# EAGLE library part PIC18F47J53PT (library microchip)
PIC18F47J53 Family High-Performance USB Microcontrollers with nanoWatt XLP Technology Source: Data sheet
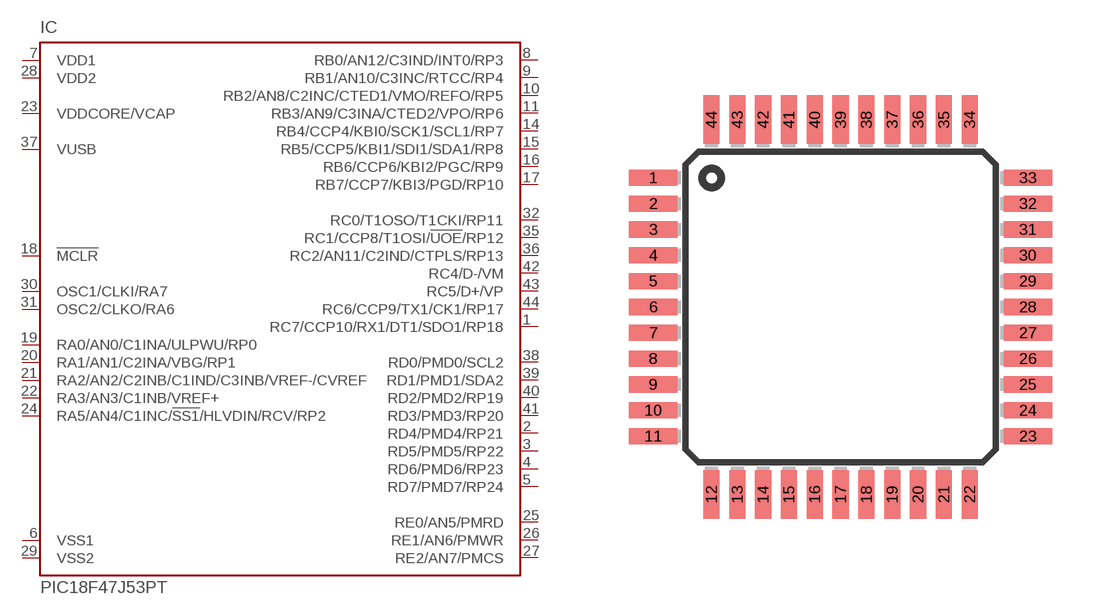
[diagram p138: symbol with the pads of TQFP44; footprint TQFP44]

Designator prefix IC

## PIC18F47J53PT (MPN: PIC18F47J53-I/PT; OC_FARNELL: 1815001; OC_NEWARK: 63R7856)  [TQFP44]
1  RC7/CCP10/RX1/DT1/SDO1/RP18
2  RD4/PMD4/RP21
3  RD5/PMD5/RP22
4  RD6/PMD6/RP23
5  RD7/PMD7/RP24
6  VSS1  in
7  VDD1  in
8  RB0/AN12/C3IND/INT0/RP3
9  RB1/AN10/C3INC/RTCC/RP4
10  RB2/AN8/C2INC/CTED1/VMO/REFO/RP5
11  RB3/AN9/C3INA/CTED2/VPO/RP6
14  RB4/CCP4/KBI0/SCK1/SCL1/RP7
15  RB5/CCP5/KBI1/SDI1/SDA1/RP8
16  RB6/CCP6/KBI2/PGC/RP9
17  RB7/CCP7/KBI3/PGD/RP10
18  !MCLR  in
19  RA0/AN0/C1INA/ULPWU/RP0
20  RA1/AN1/C2INA/VBG/RP1
21  RA2/AN2/C2INB/C1IND/C3INB/VREF-/CVREF
22  RA3/AN3/C1INB/VREF+
23  VDDCORE/VCAP  in
24  RA5/AN4/C1INC/!SS1!/HLVDIN/RCV/RP2
25  RE0/AN5/PMRD
26  RE1/AN6/PMWR
27  RE2/AN7/PMCS
28  VDD2  in
29  VSS2  in
30  OSC1/CLKI/RA7
31  OSC2/CLKO/RA6
32  RC0/T1OSO/T1CKI/RP11
35  RC1/CCP8/T1OSI/!UOE!/RP12
36  RC2/AN11/C2IND/CTPLS/RP13
37  VUSB  in
38  RD0/PMD0/SCL2
39  RD1/PMD1/SDA2
40  RD2/PMD2/RP19
41  RD3/PMD3/RP20
42  RC4/D-/VM
43  RC5/D+/VP
44  RC6/CCP9/TX1/CK1/RP17

## Footprint TQFP44 (pad centres in mm)
Thin Quad Flat Pack package type TQ
smd 1.5 x 0.5: 1 -5.8,4; 2 -5.8,3.2; 3 -5.8,2.4; 4 -5.8,1.6; 5 -5.8,0.8; 6 -5.8,0; 7 -5.8,-0.8; 8 -5.8,-1.6; 9 -5.8,-2.4; 10 -5.8,-3.2; 11 -5.8,-4; 23 5.8,-4; 24 5.8,-3.2; 25 5.8,-2.4; 26 5.8,-1.6; 27 5.8,-0.8; 28 5.8,0; 29 5.8,0.8; 30 5.8,1.6; 31 5.8,2.4; 32 5.8,3.2; 33 5.8,4
smd 0.5 x 1.5: 12 -4,-5.8; 13 -3.2,-5.8; 14 -2.4,-5.8; 15 -1.6,-5.8; 16 -0.8,-5.8; 17 0,-5.8; 18 0.8,-5.8; 19 1.6,-5.8; 20 2.4,-5.8; 21 3.2,-5.8; 22 4,-5.8; 34 4,5.8; 35 3.2,5.8; 36 2.4,5.8; 37 1.6,5.8; 38 0.8,5.8; 39 0,5.8; 40 -0.8,5.8; 41 -1.6,5.8; 42 -2.4,5.8; 43 -3.2,5.8; 44 -4,5.8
